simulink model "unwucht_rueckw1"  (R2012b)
settings: Solver=ode45  StartTime=0.0  StopTime=10.0  RelTol=1e-3
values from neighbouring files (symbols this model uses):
  c = 2200    [coulomb_1.m]    (also in coulomb_10.m = 0.1; coulomb_11.m = 0; coulomb_2.m; coulomb_3.m)
  cj = 10    [gleichstrom_motor_1.m]    (also in unwucht_rueckw_1.m = 0.1)
  g = 9.89    [foerd_gleit_1.m]    (also in foerder_haft_gleit_1.m; foerder_haft_gleit_2.m; foerderband_1.m; position_reg_1.m)
  J = 10    [gleichstrom_motor_1.m]    (also in unwucht_rueckw_1.m)
  kf = 2000    [unwucht_rueckw_1.m]    (also in vibration_control_1.m = 10; vibration_control_2.m = 10; vibration_control_3.m = 10)
  km = 10    [gleichstrom_motor_1.m]    (also in unwucht_rueckw_1.m)
  L = 1    [gleichstrom_motor_1.m]    (also in suspension_1.m = 3; suspension_2.m = 3; suspension_3.m = 3; suspension_4.m = 3)
  m = 400    [coulomb_1.m]    (also in coulomb_10.m = 10; coulomb_11.m = 10; coulomb_2.m; coulomb_3.m)
  m0 = 1    [unwucht_1.m]    (also in unwucht_2.m; unwucht_3.m; unwucht_4.m; unwucht_5.m)
  m0e = 1    [unwucht_rueckw_1.m]
  R = 0.1    [gleichstrom_motor_1.m]    (also in unwucht_rueckw_1.m; vibration_control_1.m = 15; vibration_control_2.m = 15; vibration_control_3.m = 15)
  U = fft(u)    [feder_masse_13.m]    (also in feder_masse_14.m; gleichstrom_motor_1.m = 100; unwucht_rueckw_1.m = 50)

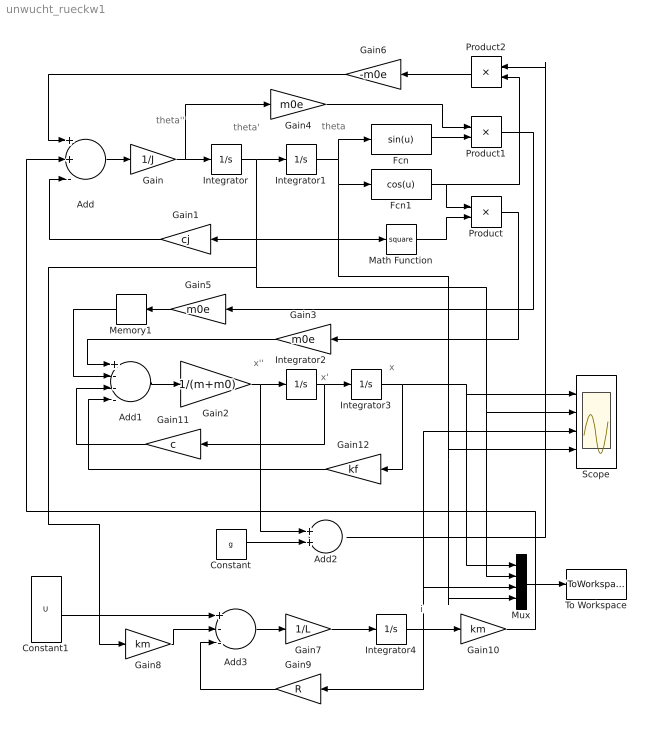
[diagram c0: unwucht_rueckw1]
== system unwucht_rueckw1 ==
  note: i
  note: x'
  note: x''
  note: theta'
  note: theta''
  note: x
  note: theta
  Add : Sum  Inputs=++-
  Add1 : Sum  Inputs=+---
  Add2 : Sum
  Add3 : Sum  Inputs=+--
  Constant : Constant  Value=g
  Constant1 : Constant  Value=U
  Fcn : Fcn  Expr=sin(u)
  Fcn1 : Fcn  Expr=cos(u)
  Gain : Gain  Gain=1/J
  Gain1 : Gain  Gain=cj
  Gain10 : Gain  Gain=km
  Gain11 : Gain  Gain=c
  Gain12 : Gain  Gain=kf
  Gain2 : Gain  Gain=1/(m+m0)
  Gain3 : Gain  Gain=m0e
  Gain4 : Gain  Gain=m0e
  Gain5 : Gain  Gain=m0e
  Gain6 : Gain  Gain=-m0e
  Gain7 : Gain  Gain=1/L
  Gain8 : Gain  Gain=km
  Gain9 : Gain  Gain=R
  Integrator{,1..4} (5 alike) : Integrator
  Math Function : Math  Operator=square
  Memory1 : Memory
  Mux : Mux
  Product : Product
  Product1 : Product
  Product2 : Product
  Scope : Scope  NumInputPorts=4
  To Workspace : ToWorkspace  VariableName=xy  SaveFormat=Structure With Time
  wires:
  Add/1 -> Gain/1
  Gain/1 -> Gain4/1, Integrator/1
  Gain1/1 -> Add/3
  Add1/1 -> Gain2/1
  Integrator2/1 -> Gain11/1, Integrator3/1
  Integrator3/1 -> Gain12/1, Mux/1, Scope/1
  Gain3/1 -> Add1/1
  Math Function/1 -> Product/2
  Product/1 -> Gain3/1
  Gain4/1 -> Product1/1
  Product1/1 -> Gain5/1
  Gain5/1 -> Memory1/1
  Constant/1 -> Add2/2
  Product2/1 -> Gain6/1
  Gain6/1 -> Add/1
  Fcn/1 -> Product1/2
  Gain7/1 -> Integrator4/1
  Add3/1 -> Gain7/1
  Constant1/1 -> Add3/1
  Gain8/1 -> Add3/2
  Gain9/1 -> Add3/3
  Gain10/1 -> Add/2
  Add2/1 -> Product2/1
  Gain11/1 -> Add1/3
  Gain12/1 -> Add1/4
  Integrator4/1 -> Gain9/1, Mux/3, Scope/3, Gain10/1
  Mux/1 -> To Workspace/1
  Integrator/1 -> Mux/2, Scope/2, Gain8/1, Math Function/1, Gain1/1, Integrator1/1
  Fcn1/1 -> Product/1, Product2/2
  Gain2/1 -> Add2/1, Integrator2/1
  Memory1/1 -> Add1/2
  Integrator1/1 -> Mux/4, Scope/4, Fcn1/1, Fcn/1
